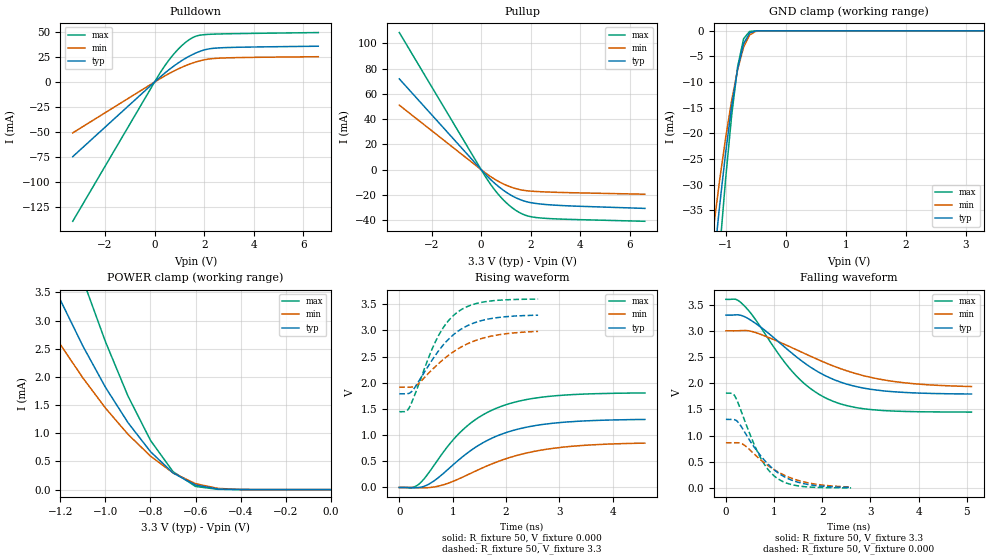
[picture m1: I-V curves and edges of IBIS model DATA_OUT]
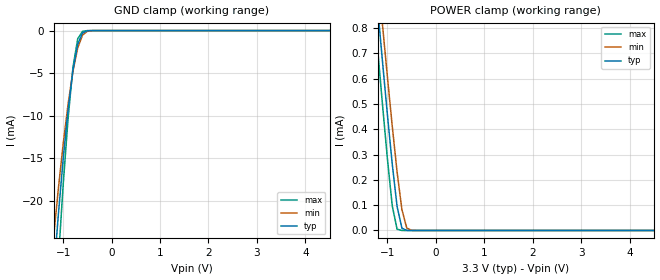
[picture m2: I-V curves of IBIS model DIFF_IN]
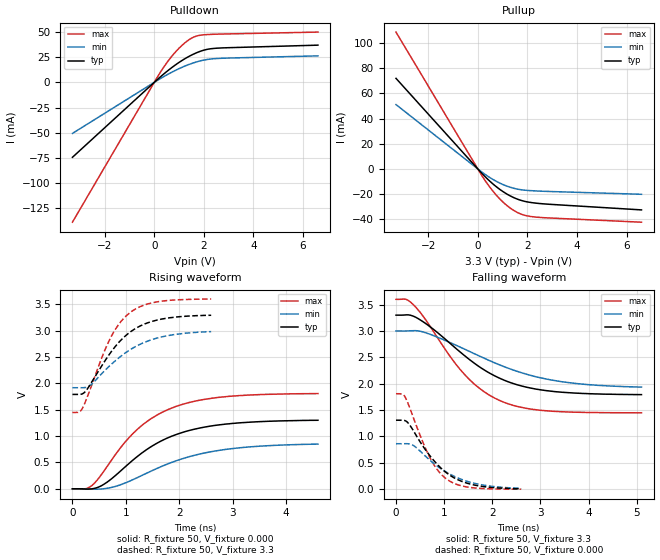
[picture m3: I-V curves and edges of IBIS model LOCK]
[IBIS ver]   3.2
[File name]   sn65lvds1224_1023.ibs
[File Rev]   0.0
[Date]   08/11/2016
[Source]   TI
[Notes]   Revision History:
| Rev 0.1: 08/11/2016
| - VQFN package pinout added for both lvds1224 and lvds1023
| Rev 0.0:  4/10/2002
| - origianl model created by PL.
[Copyright]   Copyright 2002 Mentor Graphics, Inc.
| COPYRIGHT(C) MENTOR GRAPHICS CORPORATION 2001 ALL
| RIGHTS RESERVED. THIS WORK CONTAINS PROPRIETARY
| INFORMATION WHICH IS THE PROPERTY OF MENTOR GRAPHICS
| CORPORATION OR ITS LICENSORS. USE OF THESE MATERIALS
| IS SUBJECT TO THE TERMS BELOW.
| USE: YOU MAY USE IBIS MODELS SOLELY FOR DEVELOPING
| PRINTED CIRCUIT BOARD DESIGNS. NO OTHER USE OR
| DISTRIBUTION OF THESE MATERIALS IS PERMITTED.
| DISCLAIMER OF WARRANTY:  UNLESS OTHERWISE AGREED
| IN WRITING, MENTOR GRAPHICS SOFTWARE AND ASSOCIATED
| FILES ARE PROVIDED "AS IS" AND WITHOUT WARRANTY.
| MENTOR GRAPHICS HAS NO OBLIGATION TO SUPPORT OR
| OTHERWISE MAINTAIN SOFTWARE.  MENTOR GRAPHICS MAKES
| NO WARRANTIES, EXPRESS OR IMPLIED WITH RESPECT TO
| SOFTWARE INCLUDING ANY WARRANTY OF MERCHANTABILITY
| OR FITNESS FOR A PARTICULAR PURPOSE.
| LIMITATION OF LIABILITY:  MENTOR GRAPHICS IS NOT LIABLE FOR
| ANY PROPERTY DAMAGE, PERSONAL INJURY, LOSS OF PROFITS,
| INTERRUPTION OF BUSINESS, OR FOR ANY OTHER SPECIAL,
| CONSEQUENTIAL OR INCIDENTAL DAMAGES, HOWEVER CAUSED,
| WHETHER FOR BREACH OF WARRANTY, CONTRACT, TORT
| (INCLUDING NEGLIGENCE), STRICT LIABILITY OR OTHERWISE. IN NO
| EVENT SHALL MENTOR GRAPHICS' LIABILITY EXCEED THE AMOUNT
| PAID FOR THE PRODUCT GIVING RISE TO THE CLAIM.
| TRADEMARKS:  THE FOLLOWING ARE REGISTERED TRADEMARKS
| OR SERVICE MARKS OF MENTOR GRAPHICS CORPORATION:
| ICX, ICX STANDARD LIBRARY, ICX PROJECT MODELING,
| AND ICX CUSTOM MODELING.  THE FOLLOWING ARE TRADEMARKS
| OR SERVICE MARKS OF MENTOR GRAPHICS CORPORATION:
| QUALITYIBIS, MODELVIEWER, AND MODELEDITOR. ALL OTHER
| BRANDS AND PRODUCT NAMES ARE TRADEMARKS OF THEIR
| RESPECTIVE OWNERS.
| COPIES:  ALL COPIES OF SOFTWARE, INCLUDING BUT NOT LIMITED
| TO ANY MODIFICATIONS, ENHANCEMENTS OR DERIVATIVE WORKS
| MUST CONTAIN ALL MENTOR GRAPHICS' NOTICES AND LEGENDS,
| INCLUDING THOSE EMBEDDED IN SOFTWARE AND THOSE AFFIXED
| TO THE SOFTWARE MEDIUM AND CONTAINER, AS RECEIVED FROM
| MENTOR GRAPHICS.
|   Component sn65lvds1224
[Component]   sn65lvds1224db
[Manufacturer]   TI
[Package]   | 28 pin SSOP
| variable   typ   min   max
R_pkg   0.0m   0.0m   0.0m
L_pkg   0.0nH   0.0nH   0.0nH
C_pkg   0.0pF   0.0pF   0.0pf
[Pin]   signal_name   model_name   R_pin   L_pin   C_pin
1   AGND   GND
2   RCLK_R/F   REN
3   REFCLK   REFCLK
4   AVCC   POWER
5   RI+   DIFF_IN
6   RI-   DIFF_IN
7   PWRDNB   REN
8   REN   REN
9   RCLK   DATA_OUT
10   LOCKB   LOCK
11   AVCC   POWER
12   AGND   GND
13   AGND   GND
14   DGND   GND
15   ROUT9   DATA_OUT
16   ROUT8   DATA_OUT
17   ROUT7   DATA_OUT
18   ROUT6   DATA_OUT
19   ROUT5   DATA_OUT
20   DGND   GND
21   DVCC   POWER
22   DGND   GND
23   DVCC   POWER
24   ROUT4   DATA_OUT
25   ROUT3   DATA_OUT
26   ROUT2   DATA_OUT
27   ROUT1   DATA_OUT
28   ROUT0   DATA_OUT
[Diff Pin]  inv_pin  vdiff   tdelay_typ  tdelay_min  tdelay_max
5   6   100mV   NA   NA   NA
[Component]   sn65lvds1224rhb
[Manufacturer]   TI
[Package]   | 32 pin VQFN
| variable   typ   min   max
R_pkg   0.0m   0.0m   0.0m
L_pkg   0.0nH   0.0nH   0.0nH
C_pkg   0.0pF   0.0pF   0.0pf
[Pin]   signal_name   model_name   R_pin   L_pin   C_pin
1   AVCC   POWER   NA   NA   NA
2   RI+   DIFF_IN   NA   NA   NA
3   RI-   DIFF_IN   NA   NA   NA
4   PWRDNB   REN   NA   NA   NA
5   REN   REN   NA   NA   NA
6   RCLK   DATA_OUT   NA   NA   NA
7   LOCKB   LOCK   NA   NA   NA
8   AVCC   POWER   NA   NA   NA
9   AVCC   POWER   NA   NA   NA
10   AGND   GND   NA   NA   NA
11   AGND   GND   NA   NA   NA
12   DGND   GND   NA   NA   NA
13   DGND   GND   NA   NA   NA
14   ROUT9   DATA_OUT   NA   NA   NA
15   ROUT8   DATA_OUT   NA   NA   NA
16   ROUT7   DATA_OUT   NA   NA   NA
17   ROUT6   DATA_OUT   NA   NA   NA
18   ROUT5   DATA_OUT   NA   NA   NA
19   DGND   GND   NA   NA   NA
20   DVCC   POWER   NA   NA   NA
21   DGND   GND   NA   NA   NA
22   DVCC   POWER   NA   NA   NA
23   ROUT4   DATA_OUT   NA   NA   NA
24   ROUT3   DATA_OUT   NA   NA   NA
25   ROUT2   DATA_OUT   NA   NA   NA
26   ROUT1   DATA_OUT   NA   NA   NA
27   ROUT0   DATA_OUT   NA   NA   NA
28   AGND   GND   NA   NA   NA
29   AGND   GND   NA   NA   NA
30   AGND   GND   NA   NA   NA
31   RCLK_R/F   REN   NA   NA   NA
32   REFCLK   REFCLK   NA   NA   NA
[Diff Pin]  inv_pin  vdiff   tdelay_typ  tdelay_min  tdelay_max
2   3   100mV   NA   NA   NA
|   Component sn654lvds1023
[Component]   sn654lvds1023db
[Manufacturer]   TI
[Package]   | 28 pin SSOP
| variable   typ   min   max
R_pkg   0.0m   0.0m   0.0m
L_pkg   0.0nH   0.0nH   0.0nH
C_pkg   0.0pF   0.0pF   0.0pf
[Pin]   signal_name   model_name   R_pin   L_pin   C_pin
1   SYNC1   DATA_IN
2   SYNC2   DATA_IN
3   DIN0   DATA_IN
4   DIN1   DATA_IN
5   DIN2   DATA_IN
6   DIN3   DATA_IN
7   DIN4   DATA_IN
8   DIN5   DATA_IN
9   DIN6   DATA_IN
10   DIN7   DATA_IN
11   DIN8   DATA_IN
12   DIN9   DATA_IN
13   TCLK_R/F   TCLK_R_F
14   TCLK   DATA_IN
15   DGND   GND
16   DGND   GND
17   AVCC   POWER
18   AGND   GND
19   DEN   DEN
20   AGND   GND
21   DO-   DIFF_OUT
22   DO+   DIFF_OUT
23   AGND   GND
24   PWRDNB   DEN
25   AGND   GND
26   AVCC   POWER
27   DVCC   POWER
28   DVCC   POWER
[Diff Pin]  inv_pin  vdiff   tdelay_typ  tdelay_min  tdelay_max
22   21   0V   NA   NA   NA
[Component]   sn654lvds1023rhb
[Manufacturer]   TI
[Package]   | 32 pin VQFN
| variable   typ   min   max
R_pkg   0.0m   0.0m   0.0m
L_pkg   0.0nH   0.0nH   0.0nH
C_pkg   0.0pF   0.0pF   0.0pf
[Pin]   signal_name   model_name   R_pin   L_pin   C_pin
1   DIN1   DATA_IN   NA   NA   NA
2   DIN2   DATA_IN   NA   NA   NA
3   DIN3   DATA_IN   NA   NA   NA
4   DIN4   DATA_IN   NA   NA   NA
5   DIN5   DATA_IN   NA   NA   NA
6   DIN6   DATA_IN   NA   NA   NA
7   DIN7   DATA_IN   NA   NA   NA
8   DIN8   DATA_IN   NA   NA   NA
9   DIN9   DATA_IN   NA   NA   NA
10   TCLK_R/F   TCLK_R_F   NA   NA   NA
11   TCLK   DATA_IN   NA   NA   NA
12   DGND   GND   NA   NA   NA
13   DGND   GND   NA   NA   NA
14   DGND   GND   NA   NA   NA
15   DGND   GND   NA   NA   NA
16   AVCC   POWER   NA   NA   NA
17   AGND   GND   NA   NA   NA
18   DEN   DEN   NA   NA   NA
19   AGND   GND   NA   NA   NA
20   DO-   DIFF_OUT   NA   NA   NA
21   DO+   DIFF_OUT   NA   NA   NA
22   AGND   GND   NA   NA   NA
23   PWRDNB   DEN   NA   NA   NA
24   AGND   GND   NA   NA   NA
25   AVCC   POWER   NA   NA   NA
26   DVCC   POWER   NA   NA   NA
27   DVCC   POWER   NA   NA   NA
28   DVCC   POWER   NA   NA   NA
29   DVCC   POWER   NA   NA   NA
30   SYNC1   DATA_IN   NA   NA   NA
31   SYNC2   DATA_IN   NA   NA   NA
32   DIN0   DATA_IN   NA   NA   NA
[Diff Pin]  inv_pin  vdiff   tdelay_typ  tdelay_min  tdelay_max
21   20   0V   NA   NA   NA
| Models and submodels in the file (9): DATA_OUT (3-state), DIFF_IN (Input), LOCK (Output), REFCLK (Input), REN (Input), DIFF_OUT (3-state), DATA_IN (Input), DEN (Input), TCLK_R_F (Input)
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|   Model DATA_OUT
| Developed by Hanan Elgohary
[Model]   DATA_OUT
Model_type   3-state
Polarity   Non-Inverting
Enable   Active-High
| Timing test loads and Vmeas values are assumed by ICX
Vmeas = 1.65V
Cref  = 10pF
Rref  = 1Mohms
Vref  = 3.3V
| C_comp values are extracted by ICX.
C_comp   17.5905pF   16.7429pF   17.5905pF
[Temperature Range]   27   85   -40
[Voltage Range]   3.3V   3.0V   3.6V
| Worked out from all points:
|   slope of the pulldown table from 0 to 0.495 V, typ, clamps not added: 46.7 ohm
|   slope of the pullup table from 0 to 0.495 V, typ, clamps not added: 49.9 ohm
|   GND clamp passes 1 mA (typ) near -0.63 V on its own axis
|   POWER clamp passes 1 mA (typ) near -0.86 V on its own axis
|   rising waveform, R_fixture 50, V_fixture 0.000: 20-80 % time 1.16ns typ, 1.35ns min, 1.06ns max; typ from 0 V to 1.3 V
|   rising waveform, R_fixture 50, V_fixture 3.3: 20-80 % time 706ps typ, 830ps min, 576ps max; typ from 1.79 V to 3.29 V
|   falling waveform, R_fixture 50, V_fixture 3.3: 20-80 % time 1.35ns typ, 1.73ns min, 1.14ns max; typ from 3.3 V to 1.79 V
|   falling waveform, R_fixture 50, V_fixture 0.000: 20-80 % time 714ps typ, 827ps min, 542ps max; typ from 1.31 V to 0.007 V
[Pulldown]
| voltage   I(typ)   I(min)   I(max)
-3.3V     -74.38mA   -50.68mA   -138.8mA
200mV     4.452mA    3.037mA    8.24mA
500mV     10.69mA    7.317mA    19.25mA
800mV     16.37mA    11.23mA    28.62mA
1V        19.81mA    13.62mA    33.95mA
1.3V      24.4mA     16.82mA    40.5mA
1.5V      27.04mA    18.67mA    43.81mA
1.7V      29.33mA    20.26mA    45.97mA
2V        31.97mA    22.12mA    47.22mA
2.4V      33.68mA    23.46mA    47.75mA
6.6V      35.69mA    25.24mA    49.3mA
[Pullup]
| voltage   I(typ)   I(min)   I(max)
-3.3V     71.91mA    51.08mA    108.6mA
200mV     -4.272mA   -3.027mA   -6.427mA
500mV     -10.02mA   -7.041mA   -14.91mA
700mV     -13.41mA   -9.356mA   -19.8mA
1.2V      -20.25mA   -13.84mA   -29.47mA
1.5V      -23.21mA   -15.6mA    -33.55mA
1.7V      -24.69mA   -16.38mA   -35.52mA
2V        -26.19mA   -17.05mA   -37.3mA
2.3V      -27.06mA   -17.42mA   -38.15mA
3.6V      -28.79mA   -18.29mA   -39.46mA
6.6V      -30.74mA   -19.5mA    -40.96mA
[GND_clamp]
| voltage   I(typ)   I(min)   I(max)
-3.3V     -353.7mA   -293.8mA   -441.5mA
-1.2V     -45.5mA    -38.28mA   -58.24mA
-1.1V     -34.12mA   -29.15mA   -42.91mA
-1V       -23.78mA   -20.88mA   -28.84mA
-900mV    -14.75mA   -13.6mA    -16.57mA
-800mV    -7.427mA   -7.555mA   -6.989mA
-700mV    -2.495mA   -3.149mA   -1.517mA
-600mV    -418.7uA   -807uA     -118.7uA
-500mV    -36.45uA   -118.3uA   -3.816uA
-400mV    -2.021uA   -12.09uA   -63.78nA
3.3V      4.621nA    185.4nA    4.02nA
[POWER_clamp]
| voltage   I(typ)   I(min)   I(max)
-3.3V     29.9mA     21.01mA    41.34mA
-1.4V     5.212mA    3.921mA    7.652mA
-1.3V     4.254mA    3.223mA    6.259mA
-1.2V     3.362mA    2.574mA    4.944mA
-1.1V     2.546mA    1.98mA     3.723mA
-1V       1.816mA    1.447mA    2.625mA
-900mV    1.189mA    982.1uA    1.661mA
-800mV    673.6uA    595uA      874.2uA
-700mV    295.4uA    297.5uA    319.2uA
-600mV    80.06uA    105.3uA    56.19uA
-500mV    10.83uA    21.22uA    4.448uA
0V        4.621nA    4.349nA    5.04nA
[Ramp]
| variable   typ   min   max
dV/dt_r 0.7794V/1.16018ns  0.50826V/1.34608ns  1.083V/1.0619ns
dV/dt_f 0.9042V/1.35421ns  0.6384V/1.73109ns  1.2912V/1.13739ns
R_load = 50
[Rising Waveform]
R_fixture = 50
V_fixture = 0.000
V_fixture_min = 0.000
V_fixture_max = 0.000
| time   V(typ)   V(min)   V(max)
0s        0V         0V         0V
230ps     -4.3mV     -601.4uV   -2.495mV
368ps     -930.3uV   -5.598mV   63.15mV
644ps     120.9mV    8.057mV    413.6mV
1.15ns    557.2mV    180.6mV    1.063V
1.472ns   797mV      333.9mV    1.328V
1.84ns    988.5mV    492.3mV    1.522V
2.254ns   1.122V     625.9mV    1.652V
2.852ns   1.224V     743.5mV    1.744V
4.6ns     1.299V     847.1mV    1.805V
[Rising Waveform]
R_fixture = 50
V_fixture = 3.3
V_fixture_min = 3.0
V_fixture_max = 3.6
| time   V(typ)   V(min)   V(max)
0s        1.789V     1.916V     1.447V
130ps     1.789V     1.916V     1.456V
182ps     1.797V     1.916V     1.516V
338ps     1.985V     1.963V     1.9V
702ps     2.563V     2.334V     2.837V
884ps     2.792V     2.495V     3.139V
1.066ns   2.959V     2.627V     3.329V
1.3ns     3.101V     2.755V     3.466V
1.612ns   3.205V     2.864V     3.548V
2.6ns     3.29V      2.98V      3.597V
[Falling Waveform]
R_fixture = 50
V_fixture = 3.3
V_fixture_min = 3.0
V_fixture_max = 3.6
| time   V(typ)   V(min)   V(max)
0s        3.3V       3V         3.6V
204ps     3.305V     3V         3.602V
357ps     3.282V     3.005V     3.5V
663ps     3.111V     2.952V     3.15V
1.428ns   2.53V      2.654V     2.172V
1.734ns   2.32V      2.524V     1.913V
2.142ns   2.109V     2.361V     1.687V
2.703ns   1.936V     2.182V     1.534V
3.366ns   1.845V     2.049V     1.472V
5.1ns     1.793V     1.936V     1.448V
[Falling Waveform]
R_fixture = 50
V_fixture = 0.000
V_fixture_min = 0.000
V_fixture_max = 0.000
| time   V(typ)   V(min)   V(max)
0s        1.308V     862.1mV    1.81V
182ps     1.302V     862.5mV    1.761V
286ps     1.217V     857.1mV    1.543V
390ps     1.065V     811.9mV    1.284V
702ps     637.7mV    551.6mV    604.4mV
858ps     470.2mV    436.9mV    371.5mV
1.04ns    317.5mV    327.5mV    200.7mV
1.274ns   184.9mV    217.9mV    87.54mV
1.612ns   82.26mV    115.9mV    25.66mV
2.6ns     7.323mV    16.46mV    692.6uV
|   Model DIFF_IN
|Developed by Ayah el_khordagy
[Model]   DIFF_IN
Model_type   Input
Polarity   Non-Inverting
| Vinl and vih from datasheet
Vinl = 0.8
Vinh = 2.0
| C_comp values are extracted by ICX.
C_comp   16pF   16pF   16pF
[Temperature Range]   27   85   -40
[Voltage Range]   3.3V   3.0V   3.6V
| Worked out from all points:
|   GND clamp passes 1 mA (typ) near -0.65 V on its own axis
|   POWER clamp passes 1 mA (typ) near -1.26 V on its own axis
[GND_clamp]
| voltage   I(typ)   I(min)   I(max)
-3.3V     -228.8mA   -189.9mA   -285.9mA
-1.2V     -28.87mA   -24.42mA   -36.73mA
-1.1V     -21.63mA   -18.58mA   -26.98mA
-1V       -15.06mA   -13.3mA    -18.09mA
-900mV    -9.344mA   -8.67mA    -10.37mA
-800mV    -4.716mA   -4.828mA   -4.377mA
-700mV    -1.596mA   -2.025mA   -961.2uA
-600mV    -272.1uA   -524.7uA   -77.86uA
-500mV    -24.44uA   -78uA      -2.797uA
-300mV    -59.25nA   -647.1nA   -1.416nA
6.6V      661.6pA    1.599nA    600pA
[POWER_clamp]
| voltage   I(typ)   I(min)   I(max)
-3.3V     5.576mA    5.561mA    5.606mA
-1.3V     1.093mA    1.226mA    938.9uA
-1.2V     877.3uA    1.017mA    714.4uA
-1.1V     664.9uA    810.3uA    494.6uA
-1V       458.2uA    608.1uA    283.8uA
-900mV    262.6uA    413uA      97.86uA
-800mV    95.01uA    231.3uA    5.024uA
-700mV    8.961uA    81.97uA    41.84nA
-600mV    229.1nA    9.657uA    1.259nA
-500mV    5.883nA    451.5nA    922.2pA
6.6V      661.6pA    722.3pA    720pA
|   Model LOCK
| Developed by Hanan Elgohary
[Model]   LOCK
Model_type   Output
Polarity   Non-Inverting
| The timing test loads and Vmeas are assumed by ICX
Vmeas = 1.65V
Cref  = 10pF
Rref  = 1Mohms
Vref  = 3.3V
| Ccomp values are extracted by ICX
C_comp   17.51206pF   17.51206pF   17.51206pF
[Temperature Range]   27   85   -40
[Voltage Range]   3.3V   3.0V   3.6V
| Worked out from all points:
|   slope of the pulldown table from 0 to 0.495 V, typ, clamps not added: 46.7 ohm
|   slope of the pullup table from 0 to 0.495 V, typ, clamps not added: 49.9 ohm
|   rising waveform, R_fixture 50, V_fixture 0.000: 20-80 % time 1.16ns typ, 1.35ns min, 1.06ns max; typ from 0 V to 1.3 V
|   rising waveform, R_fixture 50, V_fixture 3.3: 20-80 % time 706ps typ, 830ps min, 576ps max; typ from 1.79 V to 3.29 V
|   falling waveform, R_fixture 50, V_fixture 3.3: 20-80 % time 1.35ns typ, 1.73ns min, 1.14ns max; typ from 3.3 V to 1.79 V
|   falling waveform, R_fixture 50, V_fixture 0.000: 20-80 % time 714ps typ, 827ps min, 542ps max; typ from 1.31 V to 0.007 V
[Pulldown]
| voltage   I(typ)   I(min)   I(max)
-3.3V     -74.38mA   -50.68mA   -138.8mA
200mV     4.452mA    3.037mA    8.24mA
500mV     10.69mA    7.317mA    19.25mA
800mV     16.37mA    11.23mA    28.62mA
1V        19.81mA    13.62mA    33.95mA
1.3V      24.4mA     16.82mA    40.5mA
1.5V      27.04mA    18.67mA    43.81mA
1.7V      29.33mA    20.26mA    45.97mA
2V        31.97mA    22.12mA    47.22mA
2.4V      33.68mA    23.46mA    47.75mA
6.6V      36.94mA    26.31mA    49.91mA
[Pullup]
| voltage   I(typ)   I(min)   I(max)
-3.3V     71.91mA    51.08mA    108.6mA
200mV     -4.272mA   -3.027mA   -6.427mA
500mV     -10.02mA   -7.041mA   -14.91mA
700mV     -13.41mA   -9.356mA   -19.8mA
1.2V      -20.25mA   -13.84mA   -29.47mA
1.7V      -24.69mA   -16.38mA   -35.52mA
2.2V      -26.82mA   -17.31mA   -37.93mA
6.6V      -32.52mA   -20.13mA   -42.28mA
[Ramp]
| variable   typ   min   max
dV/dt_r 0.7794V/1.16018ns  0.50826V/1.34608ns  1.083V/1.0619ns
dV/dt_f 0.9042V/1.35421ns  0.6384V/1.73109ns  1.2912V/1.13739ns
R_load = 50
[Rising Waveform]
R_fixture = 50
V_fixture = 0.000
V_fixture_min = 0.000
V_fixture_max = 0.000
| time   V(typ)   V(min)   V(max)
0s        0V         0V         0V
230ps     -4.3mV     -601.4uV   -2.495mV
368ps     -930.3uV   -5.598mV   63.15mV
644ps     120.9mV    8.057mV    413.6mV
1.15ns    557.2mV    180.6mV    1.063V
1.472ns   797mV      333.9mV    1.328V
1.84ns    988.5mV    492.3mV    1.522V
2.254ns   1.122V     625.9mV    1.652V
2.852ns   1.224V     743.5mV    1.744V
4.6ns     1.299V     847.1mV    1.805V
[Rising Waveform]
R_fixture = 50
V_fixture = 3.3
V_fixture_min = 3.0
V_fixture_max = 3.6
| time   V(typ)   V(min)   V(max)
0s        1.789V     1.916V     1.447V
130ps     1.789V     1.916V     1.456V
182ps     1.797V     1.916V     1.516V
338ps     1.985V     1.963V     1.9V
702ps     2.563V     2.334V     2.837V
884ps     2.792V     2.495V     3.139V
1.066ns   2.959V     2.627V     3.329V
1.3ns     3.101V     2.755V     3.466V
1.612ns   3.205V     2.864V     3.548V
2.6ns     3.29V      2.98V      3.597V
[Falling Waveform]
R_fixture = 50
V_fixture = 3.3
V_fixture_min = 3.0
V_fixture_max = 3.6
| time   V(typ)   V(min)   V(max)
0s        3.3V       3V         3.6V
204ps     3.305V     3V         3.602V
357ps     3.282V     3.005V     3.5V
663ps     3.111V     2.952V     3.15V
1.428ns   2.53V      2.654V     2.172V
1.734ns   2.32V      2.524V     1.913V
2.142ns   2.109V     2.361V     1.687V
2.703ns   1.936V     2.182V     1.534V
3.366ns   1.845V     2.049V     1.472V
5.1ns     1.793V     1.936V     1.448V
[Falling Waveform]
R_fixture = 50
V_fixture = 0.000
V_fixture_min = 0.000
V_fixture_max = 0.000
| time   V(typ)   V(min)   V(max)
0s        1.308V     862.1mV    1.81V
182ps     1.302V     862.5mV    1.761V
286ps     1.217V     857.1mV    1.543V
390ps     1.065V     811.9mV    1.284V
702ps     637.7mV    551.6mV    604.4mV
858ps     470.2mV    436.9mV    371.5mV
1.04ns    317.5mV    327.5mV    200.7mV
1.274ns   184.9mV    217.9mV    87.54mV
1.612ns   82.26mV    115.9mV    25.66mV
2.6ns     7.323mV    16.46mV    692.6uV
